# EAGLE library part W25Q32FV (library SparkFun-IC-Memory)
W25Q32FV 32Mb (4MB) Serial Flash Memory The W25Q32FV support the standard Serial Peripheral Interface (SPI), Dual/Quad I/O SPI as well as 2-clocks instruction cycle Quad Peripheral Interface (QPI). 104MHz, SPI, 8-SOIC-EIAJ Datasheet SparkFun Products SparkFun Blynk Board - ESP8266 (WRL-13794)
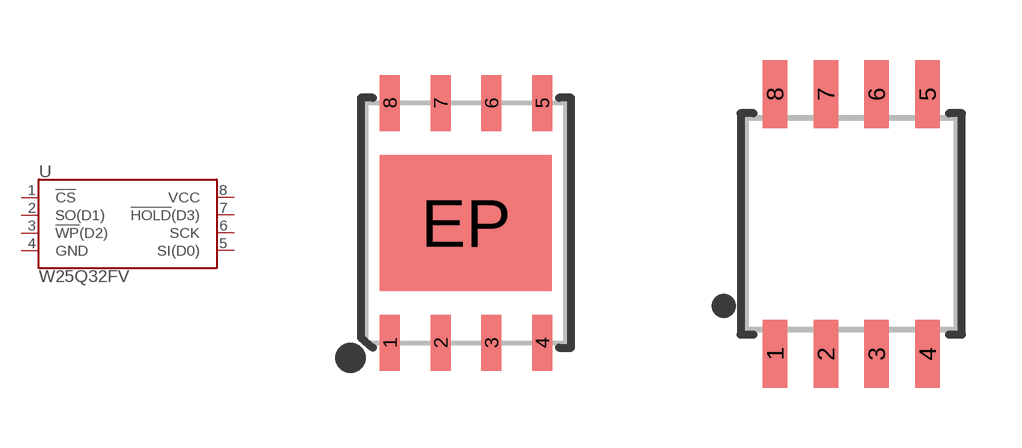
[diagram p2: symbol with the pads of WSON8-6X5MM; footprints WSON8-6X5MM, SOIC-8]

Designator prefix U

## W25Q32FVZP (PROD_ID: NA-XXXXX; VALUE: W25Q32FV)  [WSON8-6X5MM]
1  !CS!
2  SO(D1)
3  !WP!(D2)
4  GND
5  SI(D0)
6  SCK
7  !HOLD!(D3)
8  VCC

## W25Q32FVSS (PROD_ID: IC-13229; VALUE: W25Q32FV)  [SOIC-8]
Pads as for WSON8-6X5MM

## Footprint WSON8-6X5MM (pad centres in mm)
smd 0.5 x 1.4: 1 -1.905,-3; 2 -0.635,-3; 3 0.635,-3; 4 1.905,-3; 5 1.905,3; 6 0.635,3; 7 -0.635,3; 8 -1.905,3
smd 4.3 x 3.4: EP 0,0

## Footprint SOIC-8 (pad centres in mm)
8-Pin SOIC 208-mil
smd 0.61 x 1.702: 1 -1.905,-3.251; 2 -0.635,-3.251; 3 0.635,-3.251; 4 1.905,-3.251; 5 1.905,3.251; 6 0.635,3.251; 7 -0.635,3.251; 8 -1.905,3.251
